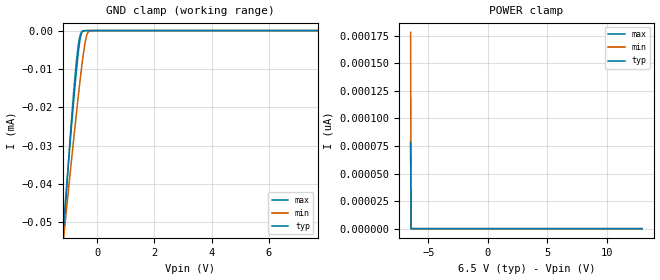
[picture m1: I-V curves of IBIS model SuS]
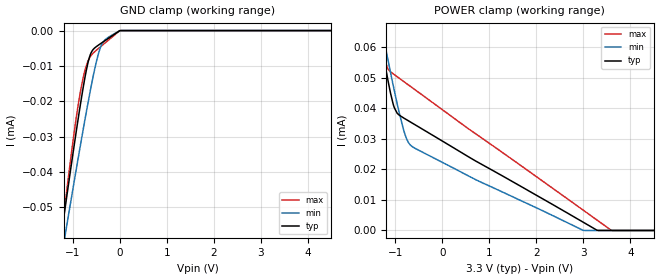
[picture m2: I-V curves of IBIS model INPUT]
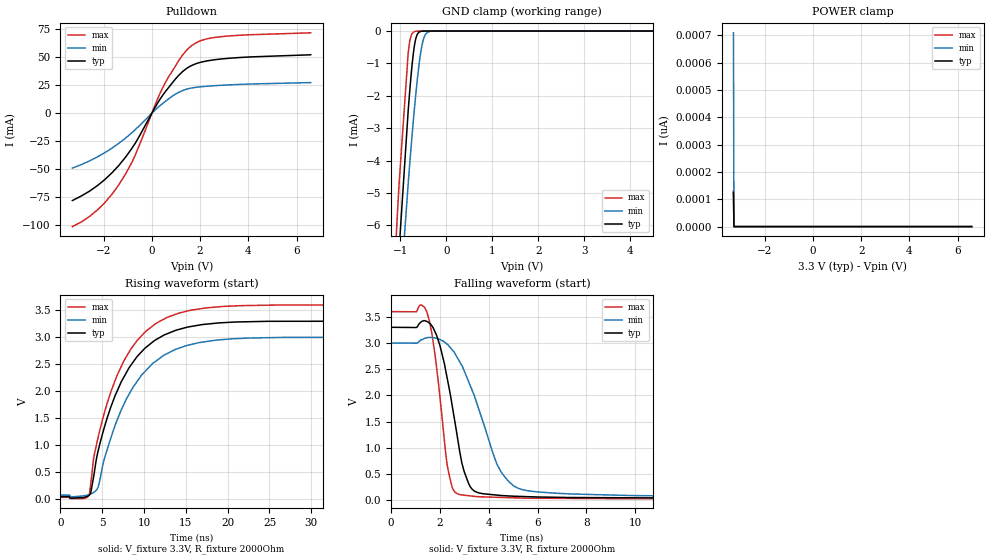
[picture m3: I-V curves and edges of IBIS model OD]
| Texas Instruments Incorporated
| Low-Noise Clock Jitter Cleaner with Dual Loop PLLs
| Marketing part#   Voltage Range   Package-type   #pins/pkg drawing
| DRV8824PWP   3.0V - 3.6V   TSSOP   28-pin PWP
| DRV8824RHD   3.0V - 3.6V   QFN   28-pin RHD
[IBIS Ver]   4.1
[File name]   drv8824.ibs
[File Rev]   0.1
[Date]   05/06/2016
[Source]   Model built from spectre simulations at:
   Texas Instruments Incorporated.
   Analog-eLab, HPA
   12500 TI Blvd
   Dallas, TX -75243
   For Support e-mail: elab_ibis@list.ti.com
[Notes]   Revision History
   Rev 0.1: 05/06/2016
   - ccomp values are based on PVT settings:
   MIN: Low Voltage, High Temperature, Weak Process
   TYP: Nominal Voltage, Nominal Temperature, Nominal Process
   MAX: High Voltage, Low Temperature, Fast Process
   - C_comp although listed in numerical order of value are obtained from varying PVT conditions.
   For PVT conditions for each specific value, refer to the buffer description under respective [Model].
   IBIS model user is responsible for using appropriate C_comp to simulate for Signal Integrity.
[Disclaimer]  This model is designed as an aid for customers of Texas Instruments
 TI and its licensors and suppliers make no warranties, either expressed
 or implied, with respect to this  model, including the warranties of
 merchantability or fitness for a particular purpose.
 The model is provided solely on an "as is" basis. The entire risk as to
 its quality and performance is with the customer.
[Copyright] (C)Copyright 2016 Texas Instruments Incorporated.
   All rights reserved.
[Component]   DRV8824PWP
[Manufacturer]  Texas Instruments Incorporated
[Package]   |28-pin PWP package
|   typ   min   max
R_pkg   0.0658   0.0227   0.1007
L_pkg   2.259E-09   1.183E-09   3.618E-09
C_pkg   3.489E-13   2.394E-13   4.969E-13
[Pin]   signal_name   model_name   R_pin   L_pin   C_pin
1   CP1   NC   0.0849   3.618E-09   4.423E-13
2   CP2   NC   0.0904   3.097E-09   4.623E-13
3   VCP   NC   0.0980   2.765E-09   3.643E-13
4   VMA   POWER   0.0361   1.900E-09   3.903E-13
5   AOUT1   NC   0.0409   1.595E-09   3.114E-13
6   ISENA   NC   0.0227   1.183E-09   3.067E-13
7   AOUT2   NC   0.0349   1.393E-09   2.768E-13
8   BOUT2   NC   0.0349   1.384E-09   2.758E-13
9   ISENB   NC   0.0227   1.183E-09   3.060E-13
10   BOUT1   NC   0.0406   1.561E-09   3.100E-13
11   VMB   POWER   0.0361   1.752E-09   3.893E-13
12   AVREF   NC   0.0983   2.680E-09   3.658E-13
13   BVREF   NC   0.0910   3.078E-09   4.619E-13
14   GND   GND   0.0345   3.159E-09   4.969E-13
15   V3P3OUT   NC   0.0819   3.512E-09   4.353E-13
16   nRESET   INPUT   0.0841   2.942E-09   4.414E-13
17   nSLEEP   INPUT   0.0878   2.495E-09   3.389E-13
18   nFAULT   OD   0.0779   2.016E-09   2.672E-13
19   DECAY   DECAY   0.0917   2.359E-09   2.806E-13
20   DIR   INPUT   0.0746   1.941E-09   2.746E-13
21   nENBL   INPUT   0.0627   1.672E-09   2.443E-13
22   STEP   INPUT   0.0609   1.589E-09   2.394E-13
23   NC   NC   0.0688   1.727E-09   2.610E-13
24   MODE0   NC   0.0836   2.073E-09   2.833E-13
25   MODE1   NC   0.1007   2.433E-09   3.054E-13
26   MODE2   NC   0.0845   2.295E-09   3.246E-13
27   nHOME   OD   0.0839   2.840E-09   4.371E-13
28   GND   GND   0.0332   3.002E-09   4.763E-13
[Component]   DRV8824RHD
[Manufacturer]  Texas Instruments Incorporated
[Package]   |28-pin RHD package
|   typ   min   max
R_pkg   0.0573   0.0200   0.0986
L_pkg   1.255E-09   6.864E-10   2.002E-09
C_pkg   2.657E-13   2.122E-13   3.807E-13
[Pin]   signal_name   model_name   R_pin   L_pin   C_pin
1   MODE2   NC   0.0672   1.270E-09   2.122E-13
2   nHOME   OD   0.0603   1.121E-09   2.223E-13
3   GND   GND   0.0200   6.864E-10   2.541E-13
4   CP1   NC   0.0544   9.977E-10   2.170E-13
5   CP2   NC   0.0572   1.064E-09   2.248E-13
6   VCP   NC   0.0667   1.265E-09   2.384E-13
7   VMA   POWER   0.0317   1.312E-09   3.151E-13
8   AOUT1   NC   0.0455   1.370E-09   3.051E-13
9   ISENA   NC   0.0277   1.035E-09   3.231E-13
10   AOUT2   NC   0.0408   1.143E-09   3.189E-13
11   BOUT2   NC   0.0413   1.140E-09   3.123E-13
12   ISENB   NC   0.0267   9.990E-10   3.118E-13
13   BOUT1   NC   0.0410   1.109E-09   3.298E-13
14   VMB   POWER   0.0346   1.297E-09   3.807E-13
15   AVREF   NC   0.0848   1.624E-09   2.513E-13
16   BVREF   NC   0.0702   1.312E-09   2.497E-13
17   GND   GND   0.0222   7.604E-10   2.795E-13
18   V3P3OUT   NC   0.0570   1.025E-09   2.225E-13
19   nRESET   INPUT   0.0542   9.896E-10   2.143E-13
20   nSLEEP   SuS   0.0577   1.057E-09   2.193E-13
21   nFAULT   OD   0.0671   1.284E-09   2.142E-13
22   DECAY   DECAY   0.0986   2.002E-09   2.714E-13
23   DIR   INPUT   0.0864   1.708E-09   2.773E-13
24   nENBL   INPUT   0.0775   1.505E-09   2.610E-13
25   STEP   INPUT   0.0729   1.420E-09   2.519E-13
26   NC   NC   0.0735   1.403E-09   2.514E-13
27   MODE0   NC   0.0785   1.521E-09   2.584E-13
28   MODE1   NC   0.0873   1.714E-09   2.503E-13
| Models and submodels in the file (4): SuS (Input), INPUT (Input), OD (Open_drain), DECAY (Output)
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|   Model SuS
[Model]   SuS
Model_type   Input
Vinl = 1.8
Vinh = 4.9
|   typ   min   max
C_comp   0.1p   0.1p   0.1p
[Voltage Range]   6.5   6   7
[Temperature Range]   27   125   -40
[Power Clamp Reference]   6.5   6   7
[GND Clamp Reference]   -0   -0   -0
[GND Clamp]
|   Voltage   I(typ)   I(min)   I(max)
-6.5V     -574.5uA   -467.6uA   -742.3uA
-1.274V   -60.05uA   -61.87uA   -66.14uA
-1.177V   -50.87uA   -54.56uA   -54.48uA
-1.157V   -49.04uA   -53.11uA   -52.18uA
-923mV    -27.53uA   -35.84uA   -26.05uA
-747.5mV  -12.45uA   -23.28uA   -9.846uA
-630.5mV  -4.092uA   -15.28uA   -2.494uA
-572mV    -1.418uA   -11.48uA   -737.3nA
-494mV    -162.8nA   -6.816uA   -72nA
-338mV    0A         -737.5nA   0A
-123.5mV  0A         0A         0A
12.98V    0A         0A         0A
[POWER Clamp]
|   Voltage   I(typ)   I(min)   I(max)
-6.5V     77.73pA    178.1pA    79.97pA
-6.461V   0A         0A         0A
-6.441V   0A         0A         0A
12.98V    0A         0A         0A
|   Model INPUT
[Model]   INPUT
Model_type   Input
Vinl = .9
Vinh = 2.52
|   typ   min   max
C_comp   0.1p   0.1p   0.1p
[Voltage Range]   3.3   3   3.6
[Temperature Range]   27   125   -40
[Power Clamp Reference]   3.3   3   3.6
[GND Clamp Reference]   -0   -0   -0
[GND Clamp]
|   Voltage   I(typ)   I(min)   I(max)
-3.3V     -258uA     -233.3uA   -305uA
-1.32V    -64.7uA    -70.29uA   -66.53uA
-1.221V   -55.35uA   -62.35uA   -55.27uA
-1.181V   -51.63uA   -59.18uA   -50.84uA
-1.112V   -45.18uA   -53.67uA   -43.21uA
-914.1mV  -27.23uA   -38.13uA   -23.28uA
-825mV    -19.63uA   -31.3uA    -16.17uA
-716.1mV  -11.35uA   -23.17uA   -9.982uA
-607.2mV  -6.136uA   -15.47uA   -6.948uA
-409.2mV  -3.678uA   -4.628uA   -4.534uA
-3.3mV    -27.83nA   -22.72nA   -35.08nA
6.59V     0A         0A         0A
[POWER Clamp]
|   Voltage   I(typ)   I(min)   I(max)
-3.3V     255.4uA    230.7uA    302.1uA
-1.468V   76.72uA    80.13uA    80.53uA
-1.33V    63.93uA    69.13uA    65.36uA
-1.31V    62.14uA    67.57uA    63.35uA
-1.27V    58.61uA    64.47uA    59.57uA
-1.171V   50.14uA    56.81uA    53.19uA
-1.023V   40.16uA    45.72uA    50.99uA
-825mV    36.82uA    32.85uA    48.77uA
-686.4mV  35.55uA    28.05uA    47.22uA
2.996V    2.719uA    24.84nA    6.672uA
3.61V     0A         0A         0A
6.59V     0A         0A         0A
|   Model OD
[Model]   OD
Model_type   Open_drain
Polarity   Non-Inverting
Vmeas = 1.65
Vref = 3.3
Cref = 15pF
Rref = 2000
|   typ   min   max
C_comp   0.738p   0.693p   0.794p
|C_comp (ON state)   0.738p   0.693p   0.794p
|C_comp (OFF state)   1.492p   1.478p   1.598p
[Voltage Range]   3.3   3   3.6
[Temperature Range]   27   125   -40
[Pullup Reference]   3.3   3   3.6
[Pulldown Reference]   -0   -0   -0
[Power Clamp Reference]   3.3   3   3.6
[GND Clamp Reference]   -0   -0   -0
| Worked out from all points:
|   slope of the pulldown table from 0 to 0.495 V, typ, clamps not added: 28.5 ohm
|   GND clamp passes 1 mA (typ) near -0.74 V on its own axis
|   falling waveform, V_fixture 3.3V, R_fixture 2000Ohm: 20-80 % time 746ps typ, 1.33ns min, 511ps max; typ from 3.3 V to 0.039 V
|   rising waveform, V_fixture 3.3V, R_fixture 2000Ohm: 20-80 % time 4.96ns typ, 5.31ns min, 4.95ns max; typ from 0.039 V to 3.3 V
[Pulldown]
|   Voltage   I(typ)   I(min)   I(max)
-3.3V     -78.41mA   -49.34mA   -101.8mA
-2.27V    -65.16mA   -39.39mA   -87.04mA
-1.924V   -59.02mA   -35.1mA    -79.56mA
-1.36V    -46.59mA   -26.89mA   -63.88mA
-706.2mV  -27.52mA   -15.16mA   -38.39mA
165mV     6.369mA    3.428mA    9.083mA
561mV     19.33mA    10.56mA    27.44mA
1.254V    36.81mA    20mA       51.45mA
1.601V    42.12mA    22.3mA     59.6mA
2.086V    45.88mA    23.69mA    65.34mA
2.779V    48.26mA    24.79mA    68.26mA
6.59V     52.25mA    27.34mA    71.95mA
[GND Clamp]
|   Voltage   I(typ)   I(min)   I(max)
-3.3V     -87.76mA   -73.56mA   -95.33mA
-1.3V     -13.99mA   -14.76mA   -12.42mA
-1.073V   -7.943mA   -9.65mA    -5.958mA
-1.023V   -6.728mA   -8.601mA   -4.69mA
-825mV    -2.436mA   -4.685mA   -654uA
-775.5mV  -1.563mA   -3.797mA   -208.4uA
-696.3mV  -505.4uA   -2.487mA   -24.43uA
-636.9mV  -130uA     -1.62mA    -4.293uA
-537.9mV  -7.682uA   -525.7uA   -135.2nA
-458.7mV  -672.9nA   -126uA     0A
-339.9mV  -35.59nA   -8.545uA   0A
6.59V     0A         0A         0A
[POWER Clamp]
|   Voltage   I(typ)   I(min)   I(max)
-3.3V     125.6pA    709.6pA    131.1pA
-3.28V    0A         0A         0A
-3.27V    0A         0A         0A
6.59V     0A         0A         0A
[Ramp]
R_load = 2000
|   typ   min   max
dV/dt_r   1.95643/4.96273e-09   1.7595/5.31051e-09   2.14422/4.955e-09
dV/dt_f   1.95643/7.46013e-10   1.7595/1.33063e-09   2.14422/5.10741e-10
[Falling Waveform]
V_fixture = 3.3V
V_fixture_min = 3V
V_fixture_max = 3.6V
R_fixture = 2000Ohm
C_fixture = 0F
|   Time   V(typ)   V(min)   V(max)
0s        3.3V       3V         3.6V
1.289ns   3.418V     3.07V      3.713V
1.72ns    3.296V     3.104V     3.037V
2.277ns   2.386V     2.986V     748.1mV
2.471ns   1.899V     2.889V     303.1mV
2.905ns   699.6mV    2.565V     97.27mV
3.47ns    158.9mV    1.909V     67.85mV
4.843ns   77.98mV    343.2mV    45.59mV
7.354ns   48.85mV    117.1mV    31.42mV
100ns     39.28mV    67.49mV    26.29mV
[Rising Waveform]
V_fixture = 3.3V
V_fixture_min = 3V
V_fixture_max = 3.6V
R_fixture = 2000Ohm
C_fixture = 0F
|   Time   V(typ)   V(min)   V(max)
0s        39.28mV    67.49mV    26.29mV
3.47ns    70.22mV    79.41mV    91.23mV
3.981ns   421.2mV    117.4mV    759.6mV
4.493ns   879.6mV    211.1mV    1.131V
5.135ns   1.263V     668.8mV    1.53V
6.736ns   1.983V     1.443V     2.277V
8.388ns   2.472V     1.991V     2.773V
11.05ns   2.913V     2.514V     3.211V
15.68ns   3.201V     2.867V     3.505V
100ns     3.3V       3V         3.6V
